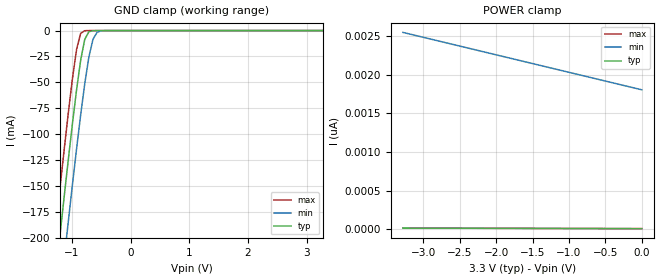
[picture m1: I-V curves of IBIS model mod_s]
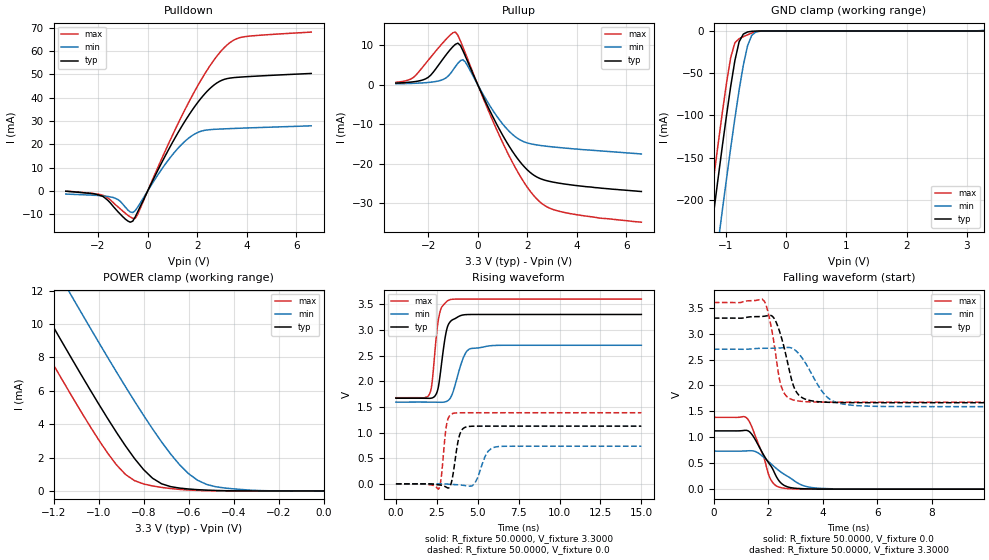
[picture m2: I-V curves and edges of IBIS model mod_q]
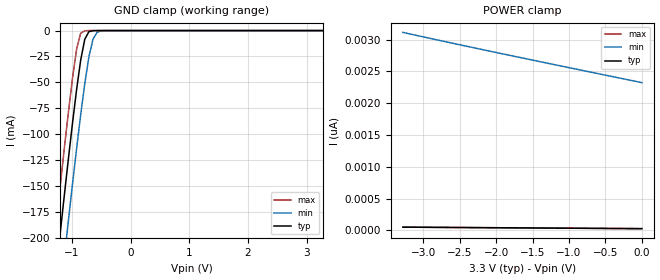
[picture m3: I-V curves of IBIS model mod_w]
| IBIS (I/O, Buffer, Information, Specification) Model, officially
| electronic behavioral standard for Buffer structures of digital pins.
[IBIS ver]  4.0
[File name] m95xxx_g8_tssop8.ibs
[File Rev]  1.0
[Date]   22 May 2015
[Source]   CAD & Design Services (Catania) - STMicroelectronics
[Notes]
   (Note1)  This IBIS model includes TSSOP8 ceramic package parasitic data
   (Note2)  This IBIS model considers: VCC=3.30(TYP), 2.70(MIN), 3.60(MAX)
   (Note3)  This IBIS model has some Notes about the non-monotonicity
   of the I-V curves, but they are not indicative of problems
   inside the model;
[Copyright] (c) 2015 STMicroelectronics
|   Component M95XXX
[Component] M95XXX
[Manufacturer] STMicroelectronics
[Package]
| variable  typ   min   max
R_pkg   0.0   0.0   0.0
L_pkg   0.0H   0.0H   0.0H
C_pkg   0.0F   0.0F   0.0F
[Pin]   signal_name   model_name   R_pin   L_pin   C_pin
1   SN   mod_s   NA   NA   NA
2   Q   mod_q   NA   NA   NA
3   WN   mod_w   NA   NA   NA
4   GND   GND   NA   NA   NA
5   D   mod_s   NA   NA   NA
6   C   mod_s   NA   NA   NA
7   HOLDN   mod_h   NA   NA   NA
8   VCC   POWER   NA   NA   NA
[Package Model]  182696_TSSOP8
[Define Package Model]  182696_TSSOP8
[Manufacturer]  STMicroelectronics
[OEM]  STMicroelectronics
[Description]  8 pin TSSOP package
[Number Of Pins]  8
[Pin Numbers]
|Pin Num   Terminal Name
1   | net1
2   | net2
3   | net3
4   | net4_GND
5   | net5
6   | net6
7   | net7
8   | net8_VDD
[Model Data]
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[End Model Data]
[End Package Model]
| Models and submodels in the file (4): mod_s (Input), mod_q (I/O), mod_w (Input), mod_h (Input)
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|   Model mod_s
[Model]   mod_s
Model_type Input
Vinl   =   1.000V
Vinh   =   2.300V
C_comp   2.120pF   2.024pF   2.323pF
[Temperature Range]  25.0000   0.1050k   -40.0000
[Voltage Range]   3.3000V   2.7000V   3.6000V
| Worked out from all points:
|   GND clamp passes 1 mA (typ) near -0.70 V on its own axis
[GND_clamp]
|Voltage   I(typ)   I(min)   I(max)
-3.3V     -1.355A    -1.412A    -1.313A
-1.34V    -270.3mA   -330.7mA   -224.8mA
-1.27V    -233mA     -293.4mA   -187.4mA
-1.2V     -196.1mA   -256.5mA   -150.5mA
-1.13V    -159.7mA   -219.9mA   -114.2mA
-1.06V    -124.1mA   -183.9mA   -79.16mA
-920mV    -57.12mA   -114.2mA   -18.15mA
-850mV    -28.51mA   -81.35mA   -2.609mA
-780mV    -8.357mA   -51.08mA   -131.1uA
-640mV    -95.71uA   -8.329mA   -224.5nA
-500mV    -655.8nA   -243.4uA   -381.5pA
3.28V     6.871pA    315.5pA    6.69pA
[POWER_clamp]
|Voltage   I(typ)   I(min)   I(max)
-3.28V    14.67pA    2.548nA    14.54pA
-1.72V    10.84pA    2.194nA    11.05pA
-920mV    8.98pA     2.013nA    9.316pA
0V        6.915pA    1.805nA    7.361pA
|   Model mod_q
[Model]   mod_q
Model_type I/O
Polarity   Non-Inverting
Enable   Active-Low
Vinl   =   1.000V
Vinh   =   2.300V
Vmeas  =   1.650V
Cref   =   30pF
C_comp   2.793pF   2.547pF   3.063pF
[Temperature Range]  25.0000   0.1050k   -40.0000
[Voltage Range]   3.3000V   2.7000V   3.6000V
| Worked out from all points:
|   slope of the pulldown table from 0 to 0.495 V, typ, clamps not added: 46.4 ohm
|   slope of the pullup table from 0 to 0.495 V, typ, clamps not added: 74.4 ohm
|   GND clamp passes 1 mA (typ) near -0.63 V on its own axis
|   POWER clamp passes 1 mA (typ) near -0.78 V on its own axis
|   rising waveform, R_fixture 50.0000, V_fixture 3.3000: 20-80 % time 433ps typ, 635ps min, 364ps max; typ from 1.67 V to 3.3 V
|   rising waveform, R_fixture 50.0000, V_fixture 0.0: 20-80 % time 337ps typ, 512ps min, 253ps max; typ from 0 V to 1.12 V
|   falling waveform, R_fixture 50.0000, V_fixture 0.0: 20-80 % time 734ps typ, 1.1ns min, 550ps max; typ from 1.12 V to 0 V
|   falling waveform, R_fixture 50.0000, V_fixture 3.3000: 20-80 % time 470ps typ, 780ps min, 362ps max; typ from 3.3 V to 1.67 V
[Pulldown]
|Voltage   I(typ)   I(min)   I(max)
-3.3V     -55uA      -1.27mA    -23uA
-1.7V     -3.1mA     -2.2mA     -2.2mA
-1.2V     -8.8mA     -3.6mA     -6.7mA
-800mV    -12.81mA   -8.05mA    -10.31mA
-600mV    -12.87mA   -9.189mA   -11.67mA
-500mV    -11.06mA   -8.352mA   -11.69mA
700mV     14.87mA    11.37mA    16.95mA
1.5V      29.85mA    21.3mA     34.77mA
2.3V      41.61mA    26.03mA    50.15mA
3V        47.52mA    26.63mA    60.44mA
3.8V      48.9mA     26.98mA    65.96mA
6.6V      50.42mA    27.98mA    68.14mA
[Pullup]
|Voltage   I(typ)   I(min)   I(max)
-3.3V     396uA      217uA      605uA
-2.6V     716uA      334uA      1.803mA
-2V       1.843mA    555uA      6.14mA
-1.3V     7.346mA    1.63mA     11.32mA
-900mV    10.2mA     4.58mA     13.29mA
-700mV    9.912mA    6.06mA     11.06mA
-500mV    7.202mA    5.732mA    7.965mA
500mV     -6.721mA   -5.43mA    -7.586mA
1.2V      -14.87mA   -11.34mA   -17.18mA
2.4V      -23.39mA   -15.25mA   -28.99mA
3.4V      -25.02mA   -15.96mA   -32.17mA
6.6V      -27mA      -17.52mA   -34.76mA
[GND_clamp]
|Voltage   I(typ)   I(min)   I(max)
-3.3V     -1.447A    -1.518A    -1.41A
-1.34V    -293.2mA   -369.8mA   -252.9mA
-1.27V    -253.6mA   -330.2mA   -213.1mA
-1.2V     -214.3mA   -291mA     -173.7mA
-1.13V    -175.5mA   -252mA     -135.1mA
-1.06V    -137.5mA   -213.6mA   -97.61mA
-920mV    -65.95mA   -139mA     -31.83mA
-780mV    -12.87mA   -70.25mA   -9.13mA
-640mV    -1.164mA   -17.66mA   -4.512mA
-570mV    -312.3uA   -5.077mA   -2.457mA
-430mV    -26.5uA    -281.9uA   -68.17uA
3.28V     150.3pA    819.4uA    122.1pA
[POWER_clamp]
|Voltage   I(typ)   I(min)   I(max)
-3.28V    60.68mA    64.24mA    58.54mA
-1.4V     14.55mA    18.3mA     12.29mA
-1.36V    13.6mA     17.35mA    11.34mA
-1.28V    11.69mA    15.45mA    9.431mA
-1.12V    7.943mA    11.69mA    5.704mA
-960mV    4.351mA    8.016mA    2.274mA
-880mV    2.694mA    6.24mA     984.9uA
-760mV    761.3uA    3.717mA    298.5uA
-600mV    115.4uA    1.036mA    55.12uA
-520mV    47.73uA    392.5uA    14.93uA
-440mV    15.03uA    175.2uA    1.974uA
0V        154.1pA    5.389nA    158pA
[Ramp]
| variable   typ   min   max
dV/dt_r  0.6746/0.3725n   0.4335/0.5753n   0.8315/0.3057n
dV/dt_f  0.9785/0.5219n   0.6458/0.8847n   1.1512/0.4317n
R_load = 50.0000
[Rising Waveform]
R_fixture= 50.0000
V_fixture= 3.3000
V_fixture_min= 2.7000   | New Temp=105 (min)
V_fixture_max= 3.6000
|time   V(typ)   V(min)   V(max)
0s        1.668V     1.592V     1.678V
2.025ns   1.666V     1.592V     1.733V
2.19ns    1.672V     1.592V     1.922V
2.49ns    1.77V      1.591V     2.939V
2.64ns    1.976V     1.59V      3.274V
3ns       2.836V     1.597V     3.518V
3.24ns    3.125V     1.638V     3.581V
4.14ns    3.292V     2.472V     3.6V
4.59ns    3.299V     2.637V     3.6V
15ns      3.3V       2.7V       3.6V
[Rising Waveform]
R_fixture= 50.0000
V_fixture= 0.0
V_fixture_min= 0.0   | New Temp = 105 (min)
V_fixture_max= 0.0
|time   V(typ)   V(min)   V(max)
0s        5.492nV    181.1nV    5.446nV
2.64ns    -20.35mV   133.7uV    -87.78mV
3.105ns   -69.88mV   -4.32mV    1.168V
3.495ns   195.2mV    -13.01mV   1.372V
3.855ns   910.2mV    -19.59mV   1.384V
4.245ns   1.104V     -35.31mV   1.385V
4.815ns   1.124V     7.329mV    1.385V
5.505ns   1.124V     567.9mV    1.385V
6.015ns   1.124V     713mV      1.385V
15ns      1.124V     733.3mV    1.385V
[Falling Waveform]
R_fixture= 50.0000
V_fixture= 0.0
V_fixture_min= 0.0   | New Temp = 105 (min)
V_fixture_max= 0.0
|time   V(typ)   V(min)   V(max)
0s        1.124V     733.3mV    1.385V
1.23ns    1.131V     739.5mV    1.361V
1.44ns    1.025V     737.7mV    1.142V
1.8ns     686.4mV    629.9mV    668mV
2.07ns    465.6mV    502.7mV    205.1mV
2.25ns    289.4mV    419mV      80.11mV
2.52ns    94.43mV    309.3mV    22.61mV
3.24ns    9.172mV    76.85mV    1.99mV
4.05ns    1.177mV    11.94mV    134.3uV
15ns      3.838nV    128.2nV    -57.47nV
[Falling Waveform]
R_fixture= 50.0000
V_fixture= 3.3000
V_fixture_min= 2.7000   | New T=105 (min)
V_fixture_max= 3.6000
|time   V(typ)   V(min)   V(max)
0s        3.3V       2.7V       3.6V
1.86ns    3.337V     2.718V     3.623V
2.19ns    3.311V     2.719V     2.881V
2.46ns    2.962V     2.725V     2.01V
2.64ns    2.598V     2.733V     1.81V
2.94ns    1.97V      2.698V     1.717V
3.27ns    1.757V     2.508V     1.691V
4.05ns    1.679V     1.835V     1.679V
4.65ns    1.671V     1.65V      1.678V
15ns      1.668V     1.592V     1.678V
|   Model mod_w
[Model]   mod_w
Model_type Input
Vinl   =   1.000V
Vinh   =   2.300V
C_comp   2.120pF   2.024pF   2.323pF
[Temperature Range]  25.0000   0.1050k   -40.0000
[Voltage Range]   3.3000V   2.7000V   3.6000V
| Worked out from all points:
|   GND clamp passes 1 mA (typ) near -0.70 V on its own axis
[GND_clamp]
|Voltage   I(typ)   I(min)   I(max)
-3.3V     -1.355A    -1.412A    -1.313A
-1.34V    -270.3mA   -330.7mA   -224.8mA
-1.27V    -233mA     -293.4mA   -187.4mA
-1.2V     -196.1mA   -256.5mA   -150.5mA
-1.13V    -159.7mA   -219.9mA   -114.2mA
-1.06V    -124.1mA   -183.9mA   -79.16mA
-920mV    -57.12mA   -114.2mA   -18.15mA
-850mV    -28.51mA   -81.35mA   -2.609mA
-780mV    -8.357mA   -51.08mA   -131.1uA
-640mV    -95.71uA   -8.329mA   -224.5nA
-500mV    -655.8nA   -243.4uA   -381.5pA
3.28V     6.871pA    315.5pA    6.69pA
[POWER_clamp]
|Voltage   I(typ)   I(min)   I(max)
-3.28V    50.17pA    3.113nA    50.46pA
-2.64V    45.35pA    2.952nA    45.72pA
-1.88V    39.76pA    2.768nA    40.16pA
0V        26.33pA    2.323nA    26.62pA
